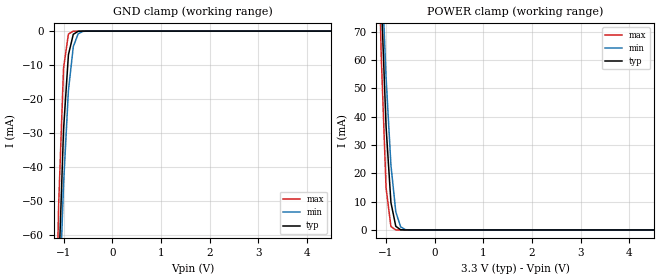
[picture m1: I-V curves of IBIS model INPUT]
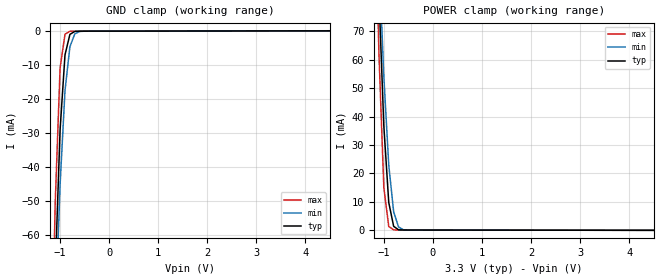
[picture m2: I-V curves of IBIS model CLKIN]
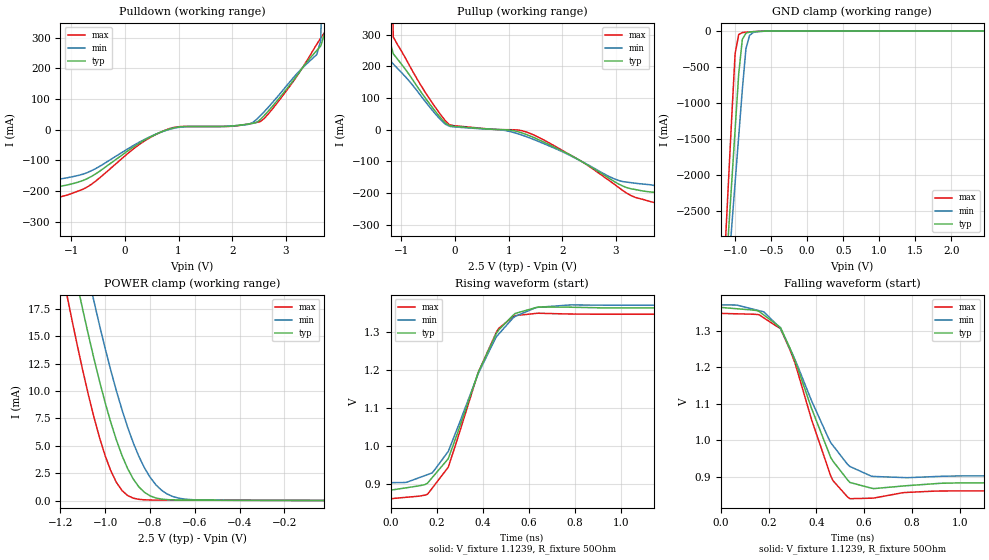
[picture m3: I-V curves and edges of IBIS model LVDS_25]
|   DIODES INCORPORATED
|   IBIS Model of PI6C5921516
|   Product Family: 6C
|   TQFN-48 Package (ZD)
[IBIS Ver] 4.0
[Comment char] |_char
[File Name] pi6c5921516_zd_reva.ibs
[File Rev] 1.0
[Source] File originated at Diodes Incorporated.
[Date] 11/16/2018
[Disclaimer] (C) Copyright DIODES INCORPORATED
   All rights reserved
 Diodes Incorporated hereby grants the user of
  this IBIS model a non-exclusive, nontransferable license to
  use this IBIS model under the following terms.
  This IBIS model is provided on an "AS IS" basis and Diodes
  makes absolutely no warranty with respect to the information
  contained herein. DIODES DISCLAIMS AND CUSTOMER WAIVES ALL
  WARRANTIES, EXPRESSED OR IMPLIED, INCLUDING WARRANTIES OF
  MERCHANTABILITY OR FITNESS FOR A PARTICULAR PURPOSE. The
  entire risk as to quality and performance is with the customer.
  Accordingly, in no event shall the company be liable for any
  damages, whether in contract or tort, including any lost
  profits or other incidental, consequential, exemplary, or
  punitive damages arising out of the use or application of the
  IBIS model provided in this package. Further, Diodes reserves
  the right to make changes without notice to any product herein
  to improve reliability, function, or design. Diodes does not
  convey any license under patent rights or any other intellectual
  property rights, including those of third parties.
  The user is granted this license only to use the IBIS model
  and is not granted rights to sell, load, rent, lease or license
  the IBIS model in whole or in part, or in modified form to anyone
  other than user. User may modify the IBIS model to suit its specific
  application but rights to derivative works and such modifications
  shall belong to Diodes.
  Diodes is not obligated to provide maintenance or support
  for the licensed IBIS model.
  Contact Diodes at ATTN: APPLICATION ENGINEERING / IBIS MODELS
  1545 Barber Ln. Milpitas, CA 95035
[Component] pi6c5912016
[Manufacturer] Diodes Incorporated.
[Package]
| variable   typ   min   max
R_pkg   0.04029ohm   NA   NA
L_pkg   2.93727nH   NA   NA
C_pkg   0.20764pF   NA   NA
[Pin]   signal_name   model_name   R_pin   L_pin   C_pin
1   GND   GND   0.04434   3.21999nH   0.24634pF
2   IN_SEL   INPUT   0.04272   3.10690nH   0.23086pF
3   REF_IN1+   CLKIN   0.04110   2.99381nH   0.21538pF
4   REF_IN1-   CLKIN   0.03948   2.88072nH   0.19990pF
5   VREF_AC1   OUTPUT   0.03786   2.76763nH   0.18442pF
6   VDD   POWER   0.03624   2.65454nH   0.16894pF
7   VDD   POWER   0.03624   2.65454nH   0.16894pF
8   VREF_AC0   OUTPUT   0.03786   2.76763nH   0.18442pF
9   REF_IN0-   CLKIN   0.03948   2.88072nH   0.19990pF
10   REF_IN0+   CLKIN   0.04110   2.99381nH   0.21538pF
11   NC   NC   0.04272   3.10690nH   0.23086pF
12   GND   GND   0.04434   3.21999nH   0.24634pF
13   VDDO   POWER   0.04434   3.21999nH   0.24634pF
14   Q0+   OUTPUT   0.04272   3.10690nH   0.23086pF
15   Q0-   OUTPUT   0.04110   2.99381nH   0.21538pF
16   Q1+   OUTPUT   0.03948   2.88072nH   0.19990pF
17   Q1-   OUTPUT   0.03786   2.76763nH   0.18442pF
18   Q2+   OUTPUT   0.03624   2.65454nH   0.16894pF
19   Q2-   OUTPUT   0.03624   2.65454nH   0.16894pF
20   Q3+   OUTPUT   0.03786   2.76763nH   0.18442pF
21   Q3-   OUTPUT   0.03948   2.88072nH   0.19990pF
22   Q4+   OUTPUT   0.04110   2.99381nH   0.21538pF
23   Q4-   OUTPUT   0.04272   3.10690nH   0.23086pF
24   VDDO   POWER   0.04434   3.21999nH   0.24634pF
25   Q5+   OUTPUT   0.04434   3.21999nH   0.24634pF
26   Q5-   OUTPUT   0.04272   3.10690nH   0.23086pF
27   Q6+   OUTPUT   0.04110   2.99381nH   0.21538pF
28   Q6-   OUTPUT   0.03948   2.88072nH   0.19990pF
29   Q7+   OUTPUT   0.03786   2.76763nH   0.18442pF
30   Q7-   OUTPUT   0.03624   2.65454nH   0.16894pF
31   Q8+   OUTPUT   0.03624   2.65454nH   0.16894pF
32   Q8-   OUTPUT   0.03786   2.76763nH   0.18442pF
33   Q9+   OUTPUT   0.03948   2.88072nH   0.19990pF
34   Q9-   OUTPUT   0.04110   2.99381nH   0.21538pF
35   Q10+   OUTPUT   0.04272   3.10690nH   0.23086pF
36   Q10-   OUTPUT   0.04434   3.21999nH   0.24634pF
37   VDDO   POWER   0.04434   3.21999nH   0.24634pF
38   Q11+   OUTPUT   0.04272   3.10690nH   0.23086pF
39   Q11-   OUTPUT   0.04110   2.99381nH   0.21538pF
40   Q12+   OUTPUT   0.03948   2.88072nH   0.19990pF
41   Q12-   OUTPUT   0.03786   2.76763nH   0.18442pF
42   Q13+   OUTPUT   0.03624   2.65454nH   0.16894pF
43   Q13-   OUTPUT   0.03624   2.65454nH   0.16894pF
44   Q14+   OUTPUT   0.03786   2.76763nH   0.18442pF
45   Q14-   OUTPUT   0.03948   2.88072nH   0.19990pF
46   Q15+   OUTPUT   0.04110   2.99381nH   0.21538pF
47   Q15-   OUTPUT   0.04272   3.10690nH   0.23086pF
48   VDDO   POWER   0.04434   3.21999nH   0.24634pF
[Diff Pin]  inv_pin vdiff   tdelay_typ tdelay_min tdelay_max
14   15   NA   0ns   0ns   0ns
16   17   NA   0ns   0ns   0ns
18   19   NA   0ns   0ns   0ns
20   21   NA   0ns   0ns   0ns
22   23   NA   0ns   0ns   0ns
25   26   NA   0ns   0ns   0ns
27   28   NA   0ns   0ns   0ns
29   30   NA   0ns   0ns   0ns
31   32   NA   0ns   0ns   0ns
33   34   NA   0ns   0ns   0ns
35   36   NA   0ns   0ns   0ns
38   39   NA   0ns   0ns   0ns
40   41   NA   0ns   0ns   0ns
42   43   NA   0ns   0ns   0ns
44   45   NA   0ns   0ns   0ns
46   47   NA   0ns   0ns   0ns
| Model DIFFOUT
[Model Selector]   OUTPUT
LVDS_33   3.3 volt VDD
LVDS_25   2.5 volt VDD
| Models and submodels in the file (4): INPUT (Input), CLKIN (Input), LVDS_25 (3-state), LVDS_33 (3-state)
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|   Model INPUT
[Model] INPUT
Model_type Input
Vinl = 800mV
Vinh = 2.00V
| variable   typ   min   max
C_comp   0.436pF   0.433pF   0.438pF
[Voltage Range]   3.300V   3.135V   3.465V
[GND Clamp Reference]   0.000V   0.000V   0.000V
[POWER Clamp Reference]  3.300V   3.135V   3.465V
[temperature range]   25   85   -40
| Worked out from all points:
|   GND clamp passes 1 mA (typ) near -0.80 V on its own axis
|   POWER clamp passes 1 mA (typ) near -0.78 V on its own axis
[GND Clamp]
| Voltage   I(typ)   I(min)   I(max)
-3.3V     -1.678A    -1.429A    -2.127A
-1.2V     -126.6mA   -133.1mA   -118.2mA
-1.1V     -71.23mA   -85.2mA    -50.81mA
-1V       -28.95mA   -45.07mA   -10.82mA
-900mV    -6.96mA    -17.47mA   -869.2uA
-800mV    -942.8uA   -4.554mA   -18.94uA
-700mV    -59.43uA   -797.7uA   -152.2nA
-600mV    -1.755uA   -80.71uA   -1.021nA
-500mV    -39.75nA   -4.639uA   -8.219pA
6.6V      19.8pA     20.38pA    19.8pA
[POWER Clamp]   |Note: Vtable = Vcc - Voutput
| Voltage   I(typ)   I(min)   I(max)
-3.3V     1.696A     1.42A      2.219A
-1.2V     140.1mA    144.7mA    134.8mA
-1.1V     82.63mA    96.09mA    62mA
-1V       36.55mA    54.02mA    14.88mA
-900mV    9.698mA    22.9mA     1.197mA
-800mV    1.302mA    6.407mA    22.02uA
-700mV    71.9uA     1.093mA    164.4nA
-600mV    1.944uA    98.92uA    1.069nA
-500mV    42.53nA    5.22uA     8.343pA
6.6V      -19.8pA    -20.38pA   -19.8pA
|   Model INPUT (CLKIN)
[Model] CLKIN
Model_type Input
Vinl = 1.20V
Vinh = 1.35V
| variable   typ   min   max
C_comp   0.483pF   0.480pF   0.486pF
[Voltage Range]   3.300V   3.135V   3.465V
[GND Clamp Reference]   0.000V   0.000V   0.000V
[POWER Clamp Reference]  3.300V   3.135V   3.465V
[temperature range]   25   85   -40
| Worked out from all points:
|   GND clamp passes 1 mA (typ) near -0.80 V on its own axis
|   POWER clamp passes 1 mA (typ) near -0.77 V on its own axis
[GND Clamp]
| Voltage   I(typ)   I(min)   I(max)
-3.3V     -1.678A    -1.429A    -2.127A
-1.2V     -126.6mA   -133.2mA   -118.2mA
-1.1V     -71.25mA   -85.22mA   -50.84mA
-1V       -28.97mA   -45.09mA   -10.85mA
-900mV    -6.977mA   -17.48mA   -892.4uA
-800mV    -958.5uA   -4.567mA   -39.57uA
-700mV    -73.12uA   -809.1uA   -18.2uA
-600mV    -13.49uA   -90.43uA   -15.47uA
-500mV    -9.82uA    -12.74uA   -12.89uA
6.6V      129.1uA    107uA      170.2uA
[POWER Clamp]   |Note: Vtable = Vcc - Voutput
| Voltage   I(typ)   I(min)   I(max)
-3.3V     1.696A     1.42A      2.22A
-1.2V     140.2mA    144.8mA    134.9mA
-1.1V     82.71mA    96.16mA    62.11mA
-1V       36.64mA    54.09mA    15mA
-900mV    9.78mA     22.96mA    1.31mA
-800mV    1.382mA    6.471mA    132uA
-700mV    150.1uA    1.155mA    107.6uA
-600mV    78.23uA    159.4uA    104.8uA
-500mV    74.37uA    64.13uA    102.3uA
6.6V      -64.55uA   -56.15uA   -80.85uA
|   Model  OUTPUT LVDS_25
[Model]  LVDS_25
Model_type  3-state
Vmeas =   1.25
| variable   typ   min   max
C_comp   2.368p   2.353p   2.489p
[Voltage Range]   2.500V   2.375V   2.625V
[GND Clamp Reference]   0.000V   0.000V   0.000V
[POWER Clamp Reference]   2.500V   2.375V   2.625V
[Pullup Reference]   2.500V   2.375V   2.625V
[Pulldown Reference]   0.000V   0.000V   0.000V
[Temperature Range]   25   85   -40
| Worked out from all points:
|   slope of the pulldown table from 0 to 0.375 V, typ, clamps not added: 8.76 ohm
|   slope of the pullup table from 0 to 0.375 V, typ, clamps not added: 72 ohm
|   GND clamp passes 1 mA (typ) near -0.52 V on its own axis
|   POWER clamp passes 1 mA (typ) near -0.84 V on its own axis
|   falling waveform, V_fixture 1.1239, R_fixture 50Ohm: 20-80 % time 165ps typ, 186ps min, 143ps max; typ from 1.36 V to 0.884 V
|   rising waveform, V_fixture 1.1239, R_fixture 50Ohm: 20-80 % time 178ps typ, 192ps min, 164ps max; typ from 0.884 V to 1.36 V
[GND Clamp]
| Voltage   I(typ)   I(min)  I(max)
-2.5V     -24.82A    -21.67A    -30.17A
-1.15V    -3.71A     -4.062A    -3.249A
-1.1V     -2.93A     -3.412A    -2.253A
-1.05V    -2.151A    -2.762A    -1.259A
-1V       -1.373A    -2.112A    -314.6mA
-950mV    -594.8mA   -1.464A    -49.05mA
-900mV    -116.6mA   -815.6mA   -21.59mA
-850mV    -30.38mA   -248.5mA   -15.67mA
-800mV    -14.44mA   -61.37mA   -12.11mA
-750mV    -9.439mA   -20.31mA   -8.857mA
-400mV    -62.11uA   -214.7uA   -5.502uA
2.45V     10.66uA    16.95uA    4.268uA
[POWER Clamp]
| Voltage   I(typ)   I(min)  I(max)
-2.5V     5.497A     4.293A     7.466A
-1.175V   24.71mA    30.57mA    19.14mA
-1.15V    22.2mA     27.9mA     16.62mA
-1.125V   19.76mA    25.32mA    14.18mA
-1.1V     17.39mA    22.84mA    11.85mA
-1.05V    12.93mA    18.16mA    7.584mA
-975mV    7.134mA    11.87mA    2.717mA
-900mV    2.929mA    6.701mA    464.9uA
-825mV    759.5uA    3.001mA    73.76uA
-750mV    145.3uA    973.1uA    47.23uA
-625mV    43.53uA    101.7uA    40.33uA
-25mV     13.86uA    14.79uA    12.46uA
[Pulldown]
| Voltage   I(typ)   I(min)  I(max)
-2.5V     -23.33A    -20.84A    -27.68A
-1.6V     -2.414A    -3.409A    -934.8mA
-1.525V   -679.6mA   -1.959A    -238.3mA
-1.45V    -198.8mA   -538.9mA   -231.1mA
-1.375V   -190.8mA   -173.9mA   -226.5mA
-700mV    -159.2mA   -139.6mA   -186.3mA
650mV     -9.226mA   -9.474mA   -9.38mA
2.375V    20.21mA    22.48mA    21.14mA
2.75V     76.33mA    88.51mA    67.81mA
3.575V    257.9mA    244.6mA    278.3mA
3.725V    317.3mA    1.116A     317.8mA
4.925V    27.57A     25.08A     33.03A
[Pullup]   |Note: Vtable = Vcc - Voutput
| Voltage   I(typ)   I(min)  I(max)
-2.425V   27.55A     21.91A     37.42A
-1.3V     1.369A     369.1mA    3.294A
-1.225V   287.8mA    222.1mA    1.064A
-175mV    20.5mA     16.85mA    27.33mA
1.4V      -19.93mA   -26.52mA   -11.73mA
3.725V    -198.2mA   -176.9mA   -230.5mA
3.8V      -199.6mA   -297.7mA   -232.6mA
3.875V    -201.3mA   -1.476A    -234.4mA
3.95V     -207.4mA   -2.925A    -236.5mA
4.025V    -680mA     -4.375A    -239mA
4.25V     -5.896A    -8.726A    -1.674A
5V        -23.32A    -23.35A    -23.96A
[Falling Waveform]
V_fixture = 1.1239
V_fixture_min = 1.1239
V_fixture_max = 1.1239
R_fixture = 50Ohm
|   Time   V(typ)   V(min)   V(max)
0s        1.364V     1.371V     1.348V
180ps     1.343V     1.352V     1.336V
250ps     1.309V     1.307V     1.306V
310ps     1.22V      1.222V     1.213V
380ps     1.087V     1.108V     1.056V
460ps     952.7mV    993.5mV    902.1mV
540ps     884.3mV    928.1mV    839.7mV
630ps     868.6mV    901.4mV    841.1mV
780ps     875.4mV    897.3mV    857mV
4ns       883.6mV    903.5mV    861.2mV
[Rising Waveform]
V_fixture = 1.1239
V_fixture_min = 1.1239
V_fixture_max = 1.1239
R_fixture = 50Ohm
|   Time   V(typ)   V(min)   V(max)
0s        883.7mV    903.5mV    861.2mV
160ps     902.2mV    924.7mV    872.8mV
180ps     916.5mV    929.2mV    888.7mV
250ps     966.7mV    985.9mV    944.4mV
380ps     1.194V     1.191V     1.194V
460ps     1.299V     1.29V      1.302V
540ps     1.35V      1.342V     1.344V
630ps     1.365V     1.365V     1.35V
780ps     1.366V     1.372V     1.348V
4ns       1.364V     1.371V     1.348V
[Ramp]
|   typ   min   max
dV/dt_r   0.27720/0.17051E-9   0.26162V/0.18235E-9   0.28558V/0.15491E-9
dV/dt_f   0.27709/0.17002E-9   0.26164V/0.18298E-9   0.28557V/0.14870E-9
R_load =   50.0000
